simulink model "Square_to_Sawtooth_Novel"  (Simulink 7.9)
settings: Solver=ode45  StartTime=0.0  StopTime=10  RelTol=3e-14
undefined symbols (not defined in the file or in its folder): sigbuilder_block
libraries: nesl_utility x6, fl_lib x5, Memristor_lib x2

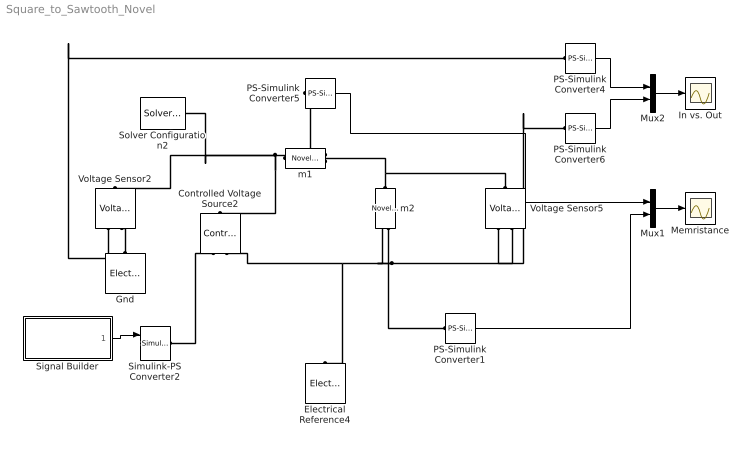
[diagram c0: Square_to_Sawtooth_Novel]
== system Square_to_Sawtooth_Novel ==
  Controlled Voltage Source2 : fl_lib/Electrical/Electrical Sources/Controlled Voltage Source  i_Log=off  v_Log=off  LocalVarNames=|i|v  LocalVarDescs=|i|v  LocalVarLogging=[0 0]
  Electrical Reference4 : fl_lib/Electrical/Electrical Elements/Electrical Reference  i_Log=off  LocalVarNames=|i  LocalVarDescs=|i  LocalVarLogging=0
  Gnd : fl_lib/Electrical/Electrical Elements/Electrical Reference  i_Log=off  LocalVarNames=|i  LocalVarDescs=|i  LocalVarLogging=0
  In vs. Out : Scope
  Memristance : Scope
  Mux1 : Mux  Inputs=2
  Mux2 : Mux  Inputs=2
  PS-Simulink Converter{1,4..6} (4 alike) : nesl_utility/PS-Simulink Converter  PhysicalDomain=network_engine_domain  LeftPortType=input  RightPortType=output  SubClassName=ps_output  Unit=1  AffineConversion=off
  Signal Builder : Subsystem  Tag=STV Subsys  LoadFcn=sigbuilder_block('load');  StartFcn=sigbuilder_block('start');  StopFcn=sigbuilder_block('stop');  ClipboardFcn=sigbuilder_block('clipboard');
  Simulink-PS Converter2 : nesl_utility/Simulink-PS Converter  PhysicalDomain=network_engine_domain  LeftPortType=input  RightPortType=output  SubClassName=ps_input  Unit=1  AffineConversion=off  InputFilterTimeConstant=.001  UdotUserProvided=2  SimscapeFilterOrder=1  InputFiltering=derivs
  Solver Configuration2 : nesl_utility/Solver Configuration  PhysicalDomain=network_engine_domain  LeftPortType=input  RightPortType=generic  SubClassName=solver  UseCustomDae=off  DoDC=off  ResidualTolerance=1e-9  UseLocalSolver=off  LocalSolverChoice=NE_BACKWARD_EULER_ADVANCER  LocalSolverSampleTime=.001  DoFixedCost=off  MaxNonlinIter=3  MaxModeIter=2  LinearAlgebra=Sparse  Accelerate=off  Profile=off  UseLocalSampling=off  DelaysMemoryBudget=1024
  Voltage Sensor2 : fl_lib/Electrical/Electrical Sensors/Voltage Sensor  i1_Log=off  v1_Log=off  LocalVarNames=|i1|v1  LocalVarDescs=|i1|v1  LocalVarLogging=[0 0]
  Voltage Sensor5 : fl_lib/Electrical/Electrical Sensors/Voltage Sensor  i1_Log=off  v1_Log=off  LocalVarNames=|i1|v1  LocalVarDescs=|i1|v1  LocalVarLogging=[0 0]
  m1 : Memristor_lib/Novel_Memristor_1  x0=5000 Ohm  M=6e3 Ohm/s  i_Log=off  v_Log=off  x_Log=off  LocalVarNames=|i|v|x  LocalVarDescs=|i|v|x  LocalVarLogging=[0 0 0]
  m2 : Memristor_lib/Novel_Memristor_1  x0=6 Ohm  M=6e3 Ohm/s  i_Log=off  v_Log=off  x_Log=off  LocalVarNames=|i|v|x  LocalVarDescs=|i|v|x  LocalVarLogging=[0 0 0]
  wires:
  Signal Builder/1(Signal 3) -> Simulink-PS Converter2/1
  Mux2/1 -> In vs. Out/1
  PS-Simulink Converter1/1 -> Mux1/2
  PS-Simulink Converter5/1 -> Mux1/1
  PS-Simulink Converter6/1 -> Mux2/2
  PS-Simulink Converter4/1 -> Mux2/1
  Mux1/1 -> Memristance/1
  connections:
  m2/LConn1 -- Voltage Sensor5/LConn1 -- m1/LConn1
  m1/RConn1 -- Solver Configuration2/RConn1 -- Controlled Voltage Source2/LConn1 -- Voltage Sensor2/LConn1
  Simulink-PS Converter2/RConn1 -- Controlled Voltage Source2/RConn1
  Voltage Sensor5/RConn2 -- Controlled Voltage Source2/RConn2 -- Electrical Reference4/LConn1 -- m2/RConn1
  Voltage Sensor5/RConn1 -- PS-Simulink Converter6/LConn1
  Voltage Sensor2/RConn1 -- PS-Simulink Converter4/LConn1
  m1/RConn2 -- PS-Simulink Converter5/LConn1
  Gnd/LConn1 -- Voltage Sensor2/RConn2
  m2/RConn2 -- PS-Simulink Converter1/LConn1

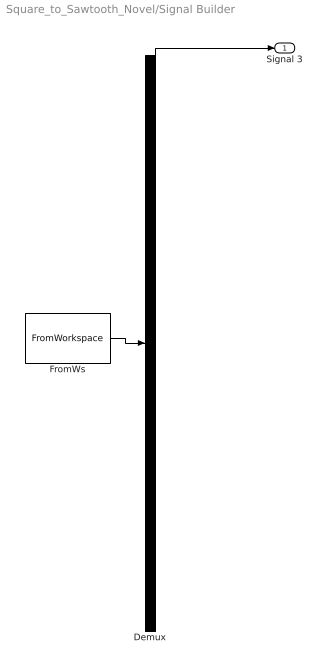
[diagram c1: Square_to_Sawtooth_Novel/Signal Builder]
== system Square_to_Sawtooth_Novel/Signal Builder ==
  Demux : Demux  Tag=STV Demux  Outputs=1
  FromWs : FromWorkspace  Tag=STV FromWs  VariableName=tuvar  SampleTime=0  SigBuilderData=DataTag0  VnvData=DataTag1
  Signal 3 : Outport  Tag=STV Outport
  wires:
  FromWs/1 -> Demux/1
  Demux/1 -> Signal 3/1
